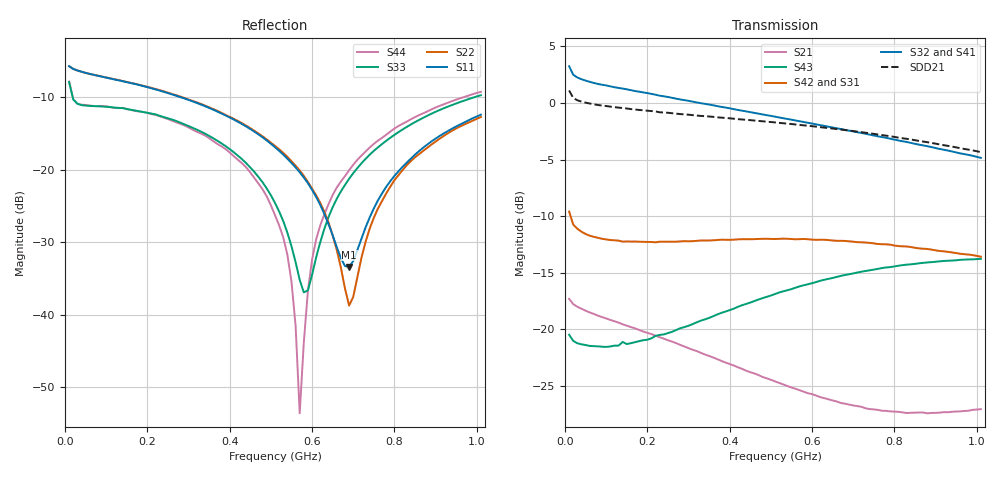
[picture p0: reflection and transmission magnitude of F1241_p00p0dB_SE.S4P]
! Integrated Device Technology
! Corporate Headquarters
! 6024 Silver Creek Valley Road
! San Jose, CA 95138  USA
! Phone:  1-408-284-8200
! Toll Free:  1-800-223-1366
! Webpage:  http://www.idt.com/
! Timing and RF Division
! 515 Groton Road, Suite 102
! Westford, MA 01886-6024
! Device:  F1241
! Description: Dual Intermediate Frequency Digital Variable Gain Amplifier
! Frequency:  10.0 -  500.00 MHz
! Package:  5x5 mm QFN Plastic Package: 32 pin
! Ports:  8 RF, 20 DC
!  Pin  1  = GA3  Pin 17  = RF OUT_B+
!  Pin  2  = GA4  Pin 18  = RF OUT_B-
!  Pin  3  = GA5  Pin 19  = STBY_B
!  Pin  4  = ISET_A  Pin 20  = Ground
!  Pin  5  = ISET_B  Pin 21  = Ground
!  Pin  6  = GB5  Pin 22  = STB_A
!  Pin  7  = GB4  Pin 23  = RF OUT_A-  = Port 4
!  Pin  8  = GB3  Pin 24  = RF OUT_A+  = Port 3
!  Pin  9  = GB2  Pin 25  = NO CONNECT
!  Pin 10  = GB1  Pin 26  = NO CONNECT
!  Pin 11  = RF IN_B+  Pin 27  = VCC
!  Pin 12  = RF IN_B-  Pin 28  = Ground
!  Pin 13  = Ground  Pin 29  = RF IN_A-  = Port 2
!  Pin 14  = VCC  Pin 30  = RF IN_A+  = Port 1
!  Pin 15  = NO CONNECT  Pin 31  = GA1
!  Pin 16  = NO CONNECT  Pin 32  = GA2
! State:  20
! Gain State:  0.0 dB
! Voltages:  Vcc = +5.00 Volts  Icc approximately 160.0 mA or 80 mA per channel.
! Data:  The device was measured on a custom evaluation board which has
!  individual transmission lines to the RF pins.  Data was collected
!  using a calibrated network analyzer.  The evaluation board was
!  de-embedded using a port reference technique.
!  The reference plane is the edge of the package pin.
!  Only Channel A was measured.
!  This data is in single-ended operation.  If your needs are balanced
!  or differential S-parameters then this file needs to be used a
!  linear simulator.
! Misc:  Lot Code  160028MY
!  Action Tracker AT004
! Date Measured:  2014-08-14
! Date:  2014-08-28  MJV
! Note:
!  Integrated Device Technology supplies this data as a sample of measured
!  data at the package pin for this product.  Your particular data for this
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# Hz S dB R 50
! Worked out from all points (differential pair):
!   101 points, 10 MHz to 1.01 GHz, reference 50 ohm
!   strongest paths, dB at 10 MHz, 260 MHz, 510 MHz, 760 MHz, 1.01 GHz:
!     S32: 3.3, 0.5, -1.2, -2.9, -4.9
!     S41: 3.3, 0.4, -1.3, -3.1, -5.1
!     S42: -9.6, -12.3, -12.0, -12.5, -13.6
!     S31: -9.6, -12.3, -12.1, -12.6, -13.7
!     S43: -20.5, -20.2, -16.9, -14.7, -13.8
!     S21: -17.3, -21.1, -24.6, -27.1, -27.1
!   taken as a pair (ports 2,1 in; 3,4 out), SDD21 dB: 1.1, -0.9, -1.7, -2.8, -4.3
!   lowest |S11| = -33.4 dB at 690 MHz (marker M1), VSWR 1.04, Z = 48.3 - j1.25 ohm
!   |S11| at or under -10 dB: 280.5 MHz to end of sweep
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1e7  -5.72 -10.0  -17.30 -14.2  -35.81 -0.6  -21.59 10.0
     -17.32 -14.1  -5.72 -9.8  -21.62 9.7  -35.87 -0.4
     -9.60 158.5  3.26 170.4  -7.91 -36.2  -20.55 -177.4
     3.30 170.5  -9.60 158.7  -20.50 -177.5  -7.85 -36.1
4.8e8  -15.55 -43.1  -24.15 -34.2  -33.57 13.4  -22.46 -27.8
       -24.23 -34.8  -15.41 -38.7  -22.27 -27.3  -33.54 11.4
       -12.10 40.5  -1.01 109.7  -21.75 -39.5  -17.44 97.1
       -1.08 108.5  -12.01 39.7  -17.25 96.8  -22.73 -31.3
5.4e8  -18.50 -49.1  -24.92 -33.2  -32.98 11.9  -22.48 -31.4
       -25.03 -33.9  -18.23 -43.1  -22.22 -31.0  -32.92 10.0
       -12.11 29.2  -1.41 102.8  -28.69 -55.0  -16.74 88.7
       -1.51 101.5  -12.01 28.1  -16.56 88.3  -31.73 -34.7
5.7e8  -20.35 -53.0  -25.27 -32.4  -32.63 11.1  -22.46 -33.3
       -25.40 -33.0  -20.12 -45.1  -22.20 -32.9  -32.61 8.7
       -12.13 23.8  -1.61 99.5  -35.21 -87.0  -16.42 84.4
       -1.72 98.1  -12.04 22.8  -16.21 84.2  -53.63 27.5
6.1e8  -23.78 -60.5  -25.72 -31.0  -32.26 10.0  -22.49 -35.9
       -25.88 -31.3  -23.56 -50.2  -22.20 -35.5  -32.19 7.8
       -12.19 17.0  -1.89 95.0  -32.09 175.9  -16.01 79.0
       -2.01 93.7  -12.10 15.7  -15.83 78.8  -29.61 137.3
6.9e8  -33.42 -142.6  -26.45 -27.1  -31.55 6.9  -22.59 -41.0
       -26.67 -27.1  -38.76 -126.6  -22.20 -40.8  -31.50 4.1
       -12.35 4.3  -2.44 86.4  -21.26 147.5  -15.34 68.4
       -2.60 85.1  -12.23 2.4  -15.14 68.0  -20.09 136.2
1.01e9  -12.41 127.4  -26.99 -8.6  -29.43 -10.8  -23.56 -60.9
        -27.07 -7.1  -12.73 127.3  -22.83 -61.4  -29.36 -13.9
        -13.73 -35.6  -4.85 55.0  -9.73 126.5  -14.00 31.6
        -5.10 53.9  -13.59 -38.8  -13.78 31.5  -9.27 122.5
